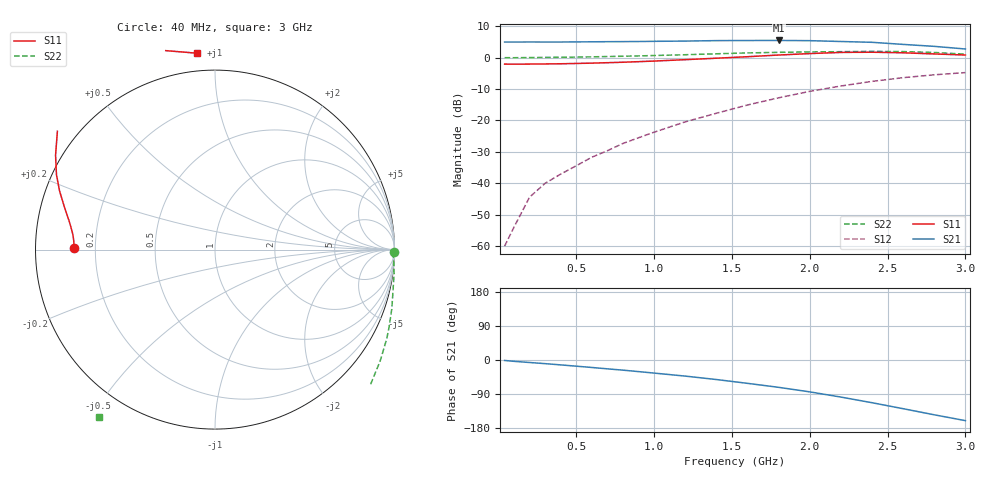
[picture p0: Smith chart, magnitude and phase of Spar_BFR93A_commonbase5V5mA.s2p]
! Filename:  BFR93ACA.S2P  Version:  2.0
! NXP part #: BFR93A  Date: Jul 1990
! Bias condition: Vce=5V, Ic=5mA
! COMMON BASE
#  MHz  S  MA  R  50
! Freq  S11  S21  S12  S22
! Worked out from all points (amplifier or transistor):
!   21 points, 40 MHz to 3 GHz, reference 50 ohm
!   highest |S21| = 5.4 dB at 1.8 GHz (marker M1)
!   |S21| within 3 dB of that: start of sweep to end of sweep
!   unconditionally stable (mu >= 1): start of sweep to 44.6 MHz
!   at 300 MHz: K = -0.48, MSG = 22.5 dB, |S12| = -40.0 dB
!   at 1 GHz: K = -0.89, MSG = 14.5 dB, |S12| = -23.7 dB
!   at 3 GHz: K = -0.43, MSG = 3.8 dB, |S12| = -4.8 dB
40  0.788 179.4  1.768 -1.2  0.001 73.1  0.996 -0.9
100  0.786 178.2  1.767 -3.5  0.002 91.5  0.995 -2.7
200  0.788 176.7  1.77 -6.6  0.006 102.8  1 -5.0
300  0.792 175.2  1.768 -9.6  0.01 112.7  1.007 -7.6
400  0.797 173.8  1.768 -12.9  0.014 121.7  1.011 -10.3
500  0.806 172.2  1.776 -16.3  0.019 127.0  1.018 -13.0
600  0.816 170.6  1.782 -19.7  0.026 129.7  1.027 -15.7
700  0.829 168.8  1.79 -23.3  0.033 132.8  1.039 -18.6
800  0.843 167.2  1.794 -26.8  0.043 134.7  1.05 -21.5
900  0.861 165.3  1.801 -30.6  0.053 136.8  1.063 -24.3
1000  0.88 163.4  1.813 -34.5  0.065 137.2  1.078 -27.4
1200  0.926 159.3  1.83 -42.5  0.095 137.4  1.11 -34.0
1400  0.977 154.7  1.861 -51.5  0.13 135.4  1.149 -41.2
1600  1.032 149.4  1.868 -61.6  0.176 132.9  1.185 -49.0
1800  1.098 143.1  1.872 -72.1  0.229 128.3  1.212 -57.9
2000  1.157 136.4  1.858 -84.1  0.29 122.5  1.231 -68.0
2200  1.208 129.5  1.802 -97.8  0.353 115.9  1.241 -79.7
2400  1.217 121.5  1.749 -112.7  0.418 107.9  1.256 -91.9
2600  1.192 113.2  1.62 -128.5  0.479 99.8  1.245 -103.4
2800  1.142 103.9  1.508 -144.6  0.532 91.4  1.206 -114.4
3000  1.099 95.3  1.369 -160.0  0.577 84.5  1.134 -124.8
